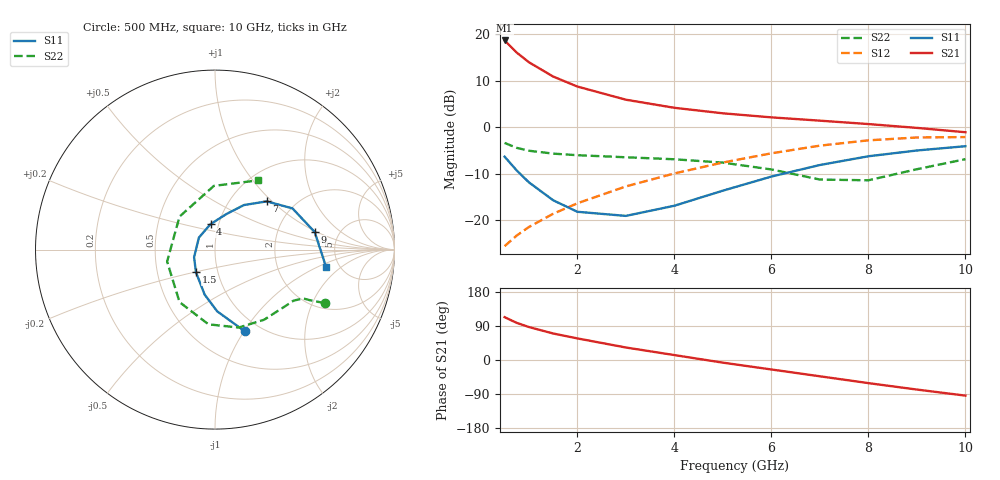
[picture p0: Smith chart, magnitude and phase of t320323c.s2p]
!AT-32032
!S-PARAMETERS at Vce=2.7V  Ic=5mA.  LAST UPDATED 05-29-98
# ghz s ma r 50
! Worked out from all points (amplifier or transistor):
!   13 points, 500 MHz to 10 GHz, reference 50 ohm
!   highest |S21| = 18.6 dB at 500 MHz (marker M1)
!   |S21| within 3 dB of that: start of sweep to 797.5 MHz
!   unconditionally stable (mu >= 1): 1.339 GHz to 3.11 GHz
!   at 1 GHz: K = 0.94, MSG = 17.7 dB, |S12| = -21.4 dB
!   at 4 GHz: K = 0.95, MSG = 7.0 dB, |S12| = -9.9 dB
!   at 10 GHz: K = 0.93, MSG = 0.5 dB, |S12| = -2.1 dB
!   lowest NFmin = 0.90 dB at 900 MHz
!   S11 on the Smith chart (normalised r, x): 500 MHz: 0.85, -1.01; 1.5 GHz: 0.78, -0.20; 4 GHz: 0.91, +0.26; 7 GHz: 1.46, +0.93; 9 GHz: 3.29, +0.95; 10 GHz: 3.93, -1.27
0.5  0.484 -70.0  8.559 113.0  0.053 62.0  0.68 -26.0
0.75  0.344 -88.0  6.339 98.0  0.069 61.0  0.602 -28.0
1  0.257 -103.0  5 87.0  0.085 61.0  0.561 -29.0
1.5  0.165 -130.0  3.509 70.0  0.118 60.0  0.522 -33.0
2  0.124 -160.0  2.74 57.0  0.153 57.0  0.502 -39.0
3  0.112 143.0  1.979 33.0  0.232 48.0  0.477 -55.0
4  0.144 100.0  1.62 13.0  0.32 37.0  0.454 -73.0
5  0.209 72.0  1.414 -7.0  0.419 24.0  0.418 -95.0
6  0.296 57.0  1.279 -25.0  0.526 8.0  0.353 -124.0
7  0.394 43.0  1.179 -43.0  0.636 -10.0  0.275 -166.0
8  0.489 28.0  1.084 -61.0  0.725 -30.0  0.27 137.0
9  0.564 10.0  0.986 -78.0  0.778 -50.0  0.355 91.0
10  0.627 -9.0  0.886 -94.0  0.786 -71.0  0.455 58.0
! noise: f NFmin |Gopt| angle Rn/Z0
0.9  0.9  0.23  71  0.15
1.8  1.2  0.295  138  0.1
2  1.2  0.31  152  0.09
2.5  1.3  0.35  -173  0.08
3  1.5  0.41  -142  0.12
3.5  1.7  0.47  -114  0.22
4  1.9  0.54  -93  0.4
